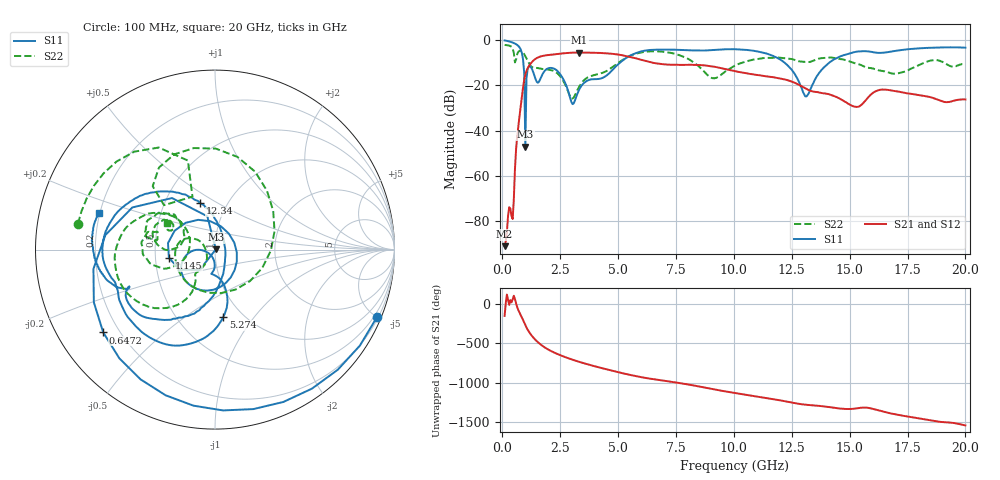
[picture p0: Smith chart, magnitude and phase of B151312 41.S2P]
!  2-Port S-parameters saved by WinCal
! VAR MeasName=S-Parameters (CALIBRATED_DATA) read from VNA (N5244A)
! VAR MeasDate=12/8/2015 5:46:55 PM
! VAR NAME=B151312 41
! VAR FILENAME=B151312 41.S2P
! VAR DATE=12/8/2015 5:46:55 PM
! VAR PHYS_PORTS=1,2
# Hz S DB R 50
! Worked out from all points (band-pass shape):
!   401 points, 100 MHz to 20 GHz, reference 50 ohm
!   highest |S21| = -5.52 dB at 3.334 GHz (marker M1); lowest = -91.0 dB at 100 MHz (marker M2)
!   |S21| within 3 dB of the highest: 1.406 GHz to 5.923 GHz (4.517 GHz wide, 123 % of centre)
!   lowest |S11| = -47.1 dB at 995.5 MHz (marker M3), VSWR 1.01, Z = 50.4 + j0.0903 ohm
!   |S11| at or under -10 dB: 908.4 MHz to 5.081 GHz (4.172 GHz wide, 139 % of centre); 12.19 GHz to 14.12 GHz (1.922 GHz wide, 14.6 % of centre)
!   |S22| runs from -25.9 to -2.2 dB; largest |S21 - S12| = 0.0022
!   S11 on the Smith chart (normalised r, x): 100 MHz: 0.29, -4.99; 647.2 MHz: 0.14, -0.32; 1.145 GHz: 0.59, -0.06; 5.274 GHz: 0.82, -0.71; 12.34 GHz: 0.75, +0.42; 20 GHz: 0.20, +0.15
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1e8  -0.20 -22.6  -90.96 -155.0  -89.93 -33.5  -2.19 169.3
3.985e8  -0.94 -87.2  -77.70 17.0  -77.13 -32.2  -3.01 129.5
6.4725e8  -2.21 -143.5  -42.26 -46.3  -42.21 -46.1  -6.11 134.5
9.955e8  -47.10 11.7  -15.26 88.9  -15.25 88.9  -7.18 48.6
1.14475e9  -11.67 -169.9  -11.58 7.2  -11.58 7.2  -10.13 -0.9
1.44325e9  -17.44 76.0  -8.25 -100.9  -8.25 -100.9  -12.31 -113.5
1.7915e9  -14.16 -72.3  -6.92 174.8  -6.92 174.8  -12.84 -163.8
2.43825e9  -14.30 -160.1  -6.10 76.7  -6.10 76.7  -15.29 159.0
3.03525e9  -28.29 -136.5  -5.58 11.6  -5.58 11.6  -25.81 -160.6
3.33375e9  -21.63 -91.2  -5.52 -16.5  -5.52 -16.4  -20.38 -125.2
3.43325e9  -19.99 -91.4  -5.53 -25.3  -5.53 -25.2  -18.83 -125.0
4.279e9  -16.90 -90.9  -5.73 -92.8  -5.73 -92.9  -14.61 -126.2
5.274e9  -8.46 -83.0  -6.92 -164.3  -6.90 -164.3  -8.30 -125.5
6.7665e9  -4.23 -131.7  -10.47 115.9  -10.47 115.8  -5.03 -175.5
9.10475e9  -4.41 -166.0  -11.71 -0.5  -11.72 -0.9  -16.87 169.1
1.005e10  -4.06 177.2  -13.74 -48.9  -13.72 -49.2  -11.25 -158.2
1.23385e10  -11.37 107.5  -17.78 -160.1  -17.83 -159.9  -8.18 166.3
1.308475e10  -24.86 19.6  -21.34 164.0  -21.34 164.3  -9.69 167.5
1.338325e10  -20.00 -58.0  -22.68 157.4  -22.66 157.3  -9.36 171.1
1.45275e10  -7.52 -115.9  -25.64 116.8  -25.60 116.4  -8.33 150.3
1.67165e10  -5.26 -156.5  -22.12 57.1  -22.02 56.6  -14.45 154.8
2e10  -3.38 162.3  -26.25 -98.5  -26.37 -99.1  -10.39 151.2
